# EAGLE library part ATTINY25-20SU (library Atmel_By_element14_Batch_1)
8-bit Microcontroller with In-System Programmable Flash
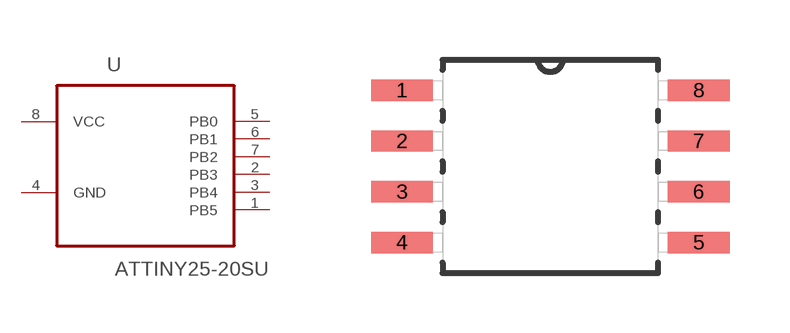
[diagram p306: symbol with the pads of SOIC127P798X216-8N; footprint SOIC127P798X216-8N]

Designator prefix U

## ATTINY25-20SU (MPN: ATTINY25-20SU; OC_FARNELL: 1455143; OC_NEWARK: 58M3779; PACKAGE: SOIC-8; SUPPLIER: Atmel)  [SOIC127P798X216-8N]
1  PB5
2  PB3
3  PB4
4  GND  pas
5  PB0
6  PB1
7  PB2
8  VCC  pwr

## Footprint SOIC127P798X216-8N (pad centres in mm)
smd 1.549 x 0.533: 1 -3.708,1.905; 2 -3.708,0.635; 3 -3.708,-0.635; 4 -3.708,-1.905; 5 3.708,-1.905; 6 3.708,-0.635; 7 3.708,0.635; 8 3.708,1.905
